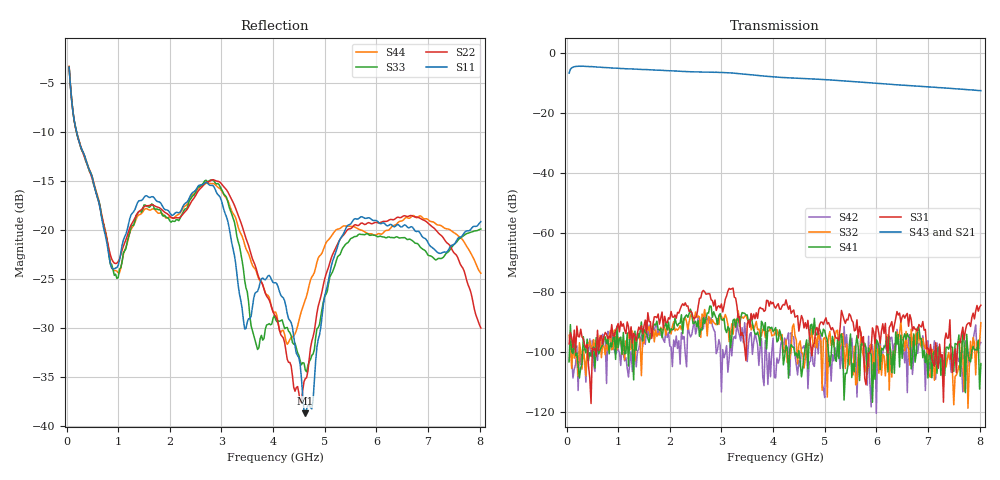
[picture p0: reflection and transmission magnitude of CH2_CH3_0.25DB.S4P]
!Agilent Technologies,E5071C,MY46316741,A.11.02
!Date: Thu May 28 14:38:17 2026
!Data & Calibration Information:
!1:CH2 INPUT 2:CH2 OUTPUT 3:CH3 INPUT 4:CH3 OUTPUT
!Freq	S11:SOLT4(ON)	S12:SOLT4(ON)	S13:SOLT4(ON)	S14:SOLT4(ON)
!	S21:SOLT4(ON)	S22:SOLT4(ON)	S23:SOLT4(ON)	S24:SOLT4(ON)
!	S31:SOLT4(ON)	S32:SOLT4(ON)	S33:SOLT4(ON)	S34:SOLT4(ON)
!	S41:SOLT4(ON)	S42:SOLT4(ON)	S43:SOLT4(ON)	S44:SOLT4(ON)
!PortZ  Port1:50+j0  Port2:50+j0  Port3:50+j0  Port4:50+j0
!Above PortZ is port z conversion or system Z0 setting when saving the data.
!When reading, reference impedance value at option line is always used.
# Hz S dB R 50
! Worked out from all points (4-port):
!   320 points, 50 MHz to 8.025 GHz, reference 50 ohm
!   strongest paths, dB at 50 MHz, 2.05 GHz, 4.05 GHz, 6.05 GHz, 8.025 GHz:
!     S43: -6.7, -5.9, -8.0, -10.2, -12.5
!     S21: -6.8, -6.1, -8.2, -10.4, -12.7
!     S31: -97.2, -88.2, -85.3, -93.9, -84.3
!     S41: -103.2, -92.5, -91.8, -98.1, -103.8
!     S32: -94.3, -91.4, -92.8, -107.0, -90.1
!     S42: -102.9, -104.8, -108.6, -102.6, -96.8
!   lowest |S11| = -38.7 dB at 4.625 GHz (marker M1), VSWR 1.02, Z = 51.1 + j0.426 ohm
!   |S11| at or under -10 dB: 195.8 MHz to end of sweep
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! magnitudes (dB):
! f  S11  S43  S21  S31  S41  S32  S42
! 50 MHz  -3.4  -6.7  -6.8  -97.2  -103.2  -94.3  -102.9
! 900 MHz  -24.0  -5.0  -5.1  -94.4  -95.6  -98.8  -98.1
! 2.825 GHz  -15.5  -6.4  -6.5  -82.7  -88.3  -89.1  -91.2
! 3.7 GHz  -26.3  -7.5  -7.7  -88.7  -93.3  -92.5  -97.5
! 4.625 GHz  -38.7  -8.5  -8.7  -90.1  -98.2  -102.3  -100.6
! 5.45 GHz  -19.5  -9.4  -9.6  -89.2  -104.5  -102.4  -103.1
! 8.025 GHz  -19.2  -12.5  -12.7  -84.3  -103.8  -90.1  -96.8
